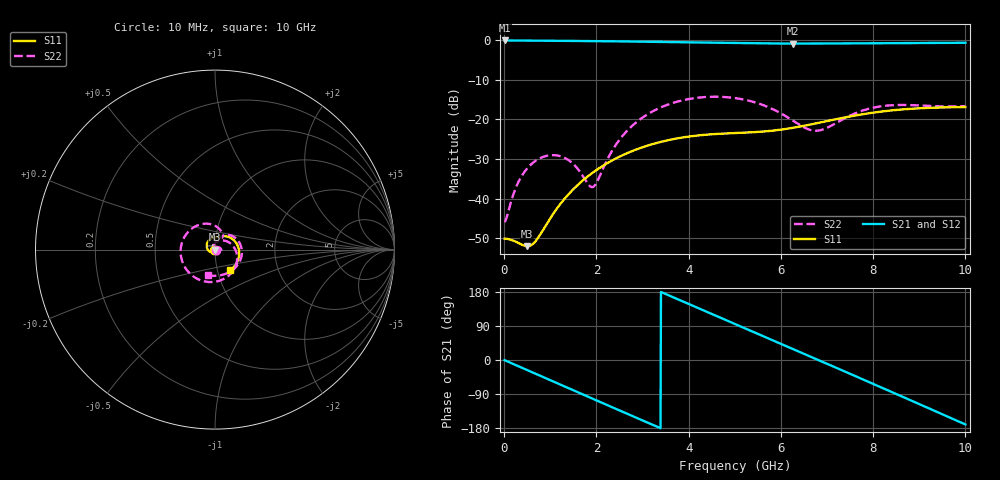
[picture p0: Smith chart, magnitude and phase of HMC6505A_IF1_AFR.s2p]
! Analog Devices, Inc.
! 1 Analog Way
! Wilmington, MA 01887
! http://www.analog.com
! Date:  2021-09-17 NN
! Board Name:  EV1HMC6505ALC5 (125487-1) with HMC6505ALC5 installed
! File Description:  Automatic Fixture Removal S-Parameters for IF1 Port connector and board loss de-embedding
! File Generation:  Calibrated Network Analyzer
! Chip Part Number:  HMC6505A
! Chip Description:  GaAs, MMIC, IQ Upconverter
! Chip Frequency:  5.5 to 8.6 GHz
! Chip Package:  LCC, 4.9 x 4.9 x 1 mm
! IF1 Port:  HMC6505ALC5 removed and end of trace left open
! Note:
!  Analog Devices supplies this data as a sample of measured data at the evaluation board
!  ports for this product.  Your particular data for this product may vary.
!  Analog Devices reserves the right to change this data at anytime.
!  All lines below in this file are as is from the Network Analyzer.
!Agilent Technologies,N5245A,MY52451809,A.10.47.06
!Automatic Fixture Removal (AFR)
!Date: Friday, September 17, 2021 3:13:00 AM
!S2P File: Measurements: S11,S21,S12,S22:
# MHz S  RI  R 50
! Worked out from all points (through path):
!   1000 points, 10 MHz to 10 GHz, reference 50 ohm
!   highest |S21| = 0.00 dB at 10 MHz (marker M1); lowest = -0.8 dB at 6.27 GHz (marker M2)
!   group delay of S21, straight-line fit = 147 ps
!   lowest |S11| = -52.1 dB at 500 MHz (marker M3), VSWR 1.01, Z = 49.8 - j0.113 ohm
!   |S11| at or under -10 dB: start of sweep to end of sweep
!   |S22| runs from -45.9 to -14.2 dB; largest |S21 - S12| = 1.4e-15
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10  -0.00311 -8.43e-06  0.9999 -0.00931  0.9999 -0.00931  0.00503 0.000434
270  -0.00279 -0.000354  0.9664 -0.2483  0.9664 -0.2483  0.0102 0.0102
500  -0.00222 -0.00114  0.8897 -0.447  0.8897 -0.447  0.0204 0.0128
690  -0.00181 -0.00231  0.7957 -0.5954  0.7957 -0.5954  0.029 0.00875
1120  -0.00244 -0.00672  0.4992 -0.8545  0.4992 -0.8545  0.0324 -0.0139
1420  -0.00531 -0.0105  0.2443 -0.9562  0.2443 -0.9562  0.0165 -0.025
1680  -0.00985 -0.0132  0.00863 -0.9844  0.00863 -0.9844  -0.0024 -0.0202
1950  -0.0164 -0.0144  -0.235 -0.9533  -0.235 -0.9533  -0.0143 0.00057
2570  -0.0347 -0.00704  -0.7083 -0.6666  -0.7083 -0.6666  0.0357 0.0511
3340  -0.0463 0.0217  -0.9577 -0.0443  -0.9577 -0.0443  0.1223 -0.0628
4080  -0.0339 0.0515  -0.7626 0.5589  -0.7626 0.5589  -0.0414 -0.18
4560  -0.018 0.0629  -0.4472 0.8234  -0.4472 0.8234  -0.1711 -0.0918
5010  -0.003 0.0673  -0.078 0.9255  -0.078 0.9255  -0.1789 0.0528
5600  0.0132 0.069  0.4057 0.8245  0.4057 0.8245  -0.0513 0.1445
6270  0.0308 0.0723  0.8023 0.4374  0.8023 0.4374  0.0402 0.087
6670  0.0451 0.0745  0.9065 0.1197  0.9065 0.1197  0.0363 0.0633
7430  0.0839 0.067  0.7722 -0.4959  0.7722 -0.4959  0.0685 0.0824
7910  0.1104 0.0468  0.4851 -0.7824  0.4851 -0.7824  0.1268 0.0518
8340  0.128 0.0174  0.143 -0.9125  0.143 -0.9125  0.1498 -0.016
9090  0.131 -0.0477  -0.4812 -0.7953  -0.4812 -0.7953  0.0894 -0.1199
9570  0.1125 -0.0872  -0.7819 -0.5088  -0.7819 -0.5088  0.0232 -0.1441
10000  0.0856 -0.1154  -0.9212 -0.161  -0.9212 -0.161  -0.0406 -0.1421
